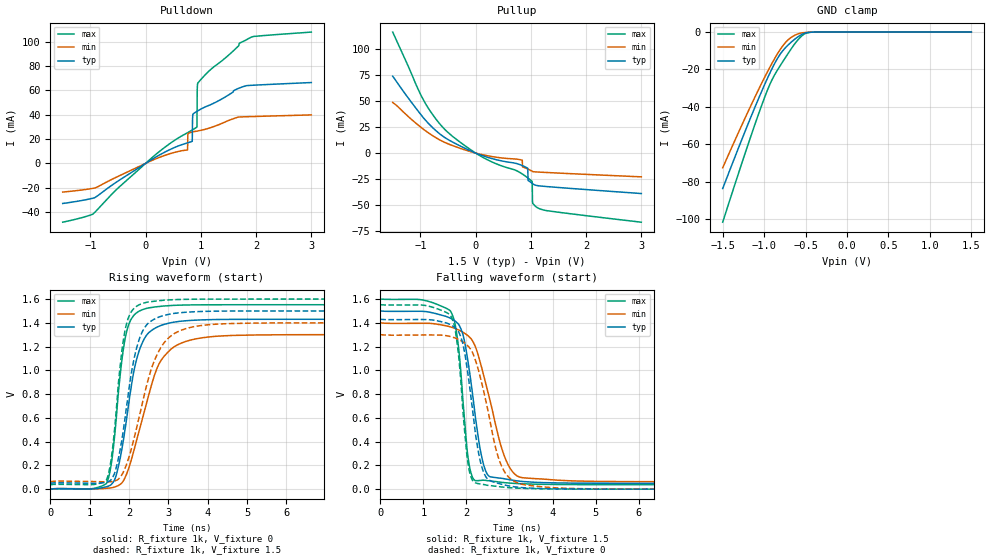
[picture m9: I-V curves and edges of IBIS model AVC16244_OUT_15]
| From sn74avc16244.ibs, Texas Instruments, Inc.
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[Model]   AVC16244_OUT_15
Model_type  3-state
Enable   Active-Low
Vref =   0
Rref =   2k
Cref =   15p
Vmeas =   0.75
| variable   typ   min   max
C_comp   4.20pF   3.38pF   5.49pF
| C_pullup   5.53pF   0.12pF   14.01pF
| C_pulldown   8.09pF   0.20pF   29.17pF
| C_tri-state   4.20pF   3.38pF   5.49pF
[Temperature Range]   40   100   -40
| Ambient temperature   25   85   -40
[Voltage range]   1.5   1.4   1.6
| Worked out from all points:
|   slope of the pulldown table from 0 to 0.225 V, typ, clamps not added: 36.1 ohm
|   slope of the pullup table from 0 to 0.225 V, typ, clamps not added: 53.5 ohm
|   GND clamp passes 1 mA (typ) near -0.53 V on its own axis
|   rising waveform, R_fixture 1k, V_fixture 0: 20-80 % time 448ps typ, 673ps min, 298ps max; typ from 0 V to 1.43 V
|   falling waveform, R_fixture 1k, V_fixture 1.5: 20-80 % time 344ps typ, 562ps min, 228ps max; typ from 1.5 V to 0.049 V
|   rising waveform, R_fixture 1k, V_fixture 1.5: 20-80 % time 434ps typ, 663ps min, 288ps max; typ from 0.049 V to 1.5 V
|   falling waveform, R_fixture 1k, V_fixture 0: 20-80 % time 332ps typ, 499ps min, 225ps max; typ from 1.43 V to 0 V
[GND Clamp]
| AVC16244_OUT_15
|   Voltage   I(typ)   I(min)   I(max)
-1.5V     -83.68mA   -72.57mA   -101.7mA
-1.15V    -44.37mA   -38.39mA   -54.38mA
-1.025V   -31.19mA   -26.93mA   -38.6mA
-940mV    -22.8mA    -19.57mA   -28.92mA
-890mV    -18.24mA   -15.49mA   -24.21mA
-830mV    -13.44mA   -10.97mA   -19.64mA
-735mV    -7.99mA    -5.222mA   -13.08mA
-645mV    -4.324mA   -2.051mA   -7.147mA
-535mV    -1.034mA   -356.6uA   -1.661mA
-485mV    -307.6uA   -164.9uA   -439.4uA
-395mV    -28.13uA   -34.37uA   -21.37uA
1.5V      921pA      11.46nA    28.98pA
[Pulldown]
| AVC16244_OUT_15
|   Voltage   I(typ)   I(min)   I(max)
-1.5V     -33mA      -23.61mA   -48.39mA
-955mV    -28.68mA   -20.56mA   -41.74mA
760mV     16.89mA    11.08mA    25.23mA
770mV     17.03mA    24.64mA    25.49mA
845mV     18.17mA    25.77mA    27.48mA
855mV     40.2mA     25.88mA    27.75mA
925mV     42.66mA    26.52mA    29.72mA
930mV     42.8mA     26.55mA    30.08mA
935mV     42.94mA    26.59mA    61.05mA
945mV     43.22mA    26.68mA    66.04mA
1.695V    61.97mA    38.15mA    98.75mA
3V        66.51mA    39.88mA    108mA
[Pullup]
| AVC16244_OUT_15
|   Voltage   I(typ)   I(min)   I(max)
-1.5V     73.5mA     48.38mA    115.7mA
-980mV    36.08mA    24.24mA    54.47mA
-665mV    19.05mA    13.02mA    28.99mA
20mV      -420.5uA   -275.9uA   -662.9uA
940mV     -14.35mA   -15.15mA   -23.58mA
950mV     -26.22mA   -15.4mA    -23.99mA
1.02V     -28.75mA   -17.27mA   -26.94mA
1.025V    -28.95mA   -17.41mA   -27.17mA
1.03V     -29.14mA   -17.56mA   -46.58mA
1.035V    -29.33mA   -17.7mA    -48.24mA
1.1V      -30.94mA   -18.07mA   -51.63mA
3V        -38.73mA   -22.77mA   -66.15mA
[Ramp]
| AVC16244_OUT_15
| variable   typ   min   max
dV/dt_r   0.86/4.55E-10   0.78/6.75E-10   0.93/3.05E-10
dV/dt_f   0.87/3.53E-10   0.80/5.68E-10   0.94/2.35E-10
R_load = 1k
[Rising Waveform]
| AVC16244_OUT_15
R_fixture =   1k
C_fixture =   0
L_fixture =   0
V_fixture =   0
V_fixture_min = 0
V_fixture_max = 0
|   Time   V(typ)   V(min)   V(max)
0s        19.89nV    104.5nV    630.1pV
1.43ns    20.42mV    7.697mV    47.95mV
1.555ns   40.98mV    11.25mV    222.4mV
1.685ns   129mV      23.94mV    628.2mV
1.825ns   347.9mV    54.32mV    1.1V
1.975ns   674.1mV    158.4mV    1.367V
2.29ns    1.193V     529.8mV    1.503V
2.825ns   1.379V     1.089V     1.539V
5.255ns   1.43V      1.298V     1.552V
50ns      1.43V      1.3V       1.552V
[Falling Waveform]
| AVC16244_OUT_15
R_fixture =   1k
C_fixture =   0
L_fixture =   0
V_fixture =   1.5
V_fixture_min = 1.4
V_fixture_max = 1.6
|   Time   V(typ)   V(min)   V(max)
0s        1.5V       1.4V       1.6V
1.645ns   1.436V     1.364V     1.489V
1.8ns     1.395V     1.343V     1.243V
1.93ns    1.286V     1.318V     698.4mV
2.06ns    1.019V     1.284V     213.8mV
2.22ns    575.7mV    1.188V     70.68mV
2.48ns    129mV      844.7mV    72.41mV
3.015ns   78.87mV    176mV      50.95mV
4.11ns    52.47mV    75.48mV    39.36mV
50ns      49.24mV    62.36mV    37.6mV
[Rising Waveform]
| AVC16244_OUT_15
R_fixture =   1k
C_fixture =   0
L_fixture =   0
V_fixture =   1.5
V_fixture_min = 1.4
V_fixture_max = 1.6
|   Time   V(typ)   V(min)   V(max)
0s        49.24mV    62.36mV    37.6mV
1.43ns    58.97mV    62.44mV    77.62mV
1.555ns   83.79mV    62.89mV    270.2mV
1.685ns   192.4mV    75.34mV    696.9mV
1.82ns    417.4mV    120.7mV    1.165V
1.965ns   757.7mV    234.5mV    1.423V
2.295ns   1.292V     658.7mV    1.557V
2.83ns    1.456V     1.202V     1.588V
5.16ns    1.5V       1.398V     1.6V
50ns      1.5V       1.4V       1.6V
[Falling Waveform]
| AVC16244_OUT_15
R_fixture =   1k
C_fixture =   0
L_fixture =   0
V_fixture =   0
V_fixture_min = 0
V_fixture_max = 0
|   Time   V(typ)   V(min)   V(max)
0s        1.43V      1.3V       1.552V
1.625ns   1.385V     1.285V     1.466V
1.79ns    1.338V     1.265V     1.214V
2.01ns    1.032V     1.214V     291.8mV
2.095ns   805.3mV    1.179V     114.2mV
2.39ns    152.1mV    841.8mV    39.88mV
2.695ns   53.32mV    324.9mV    23.81mV
2.925ns   31.89mV    124.8mV    14.67mV
5.17ns    427.4uV    1.858mV    195.4uV
50ns      19.31nV    99.52nV    13.01nV
